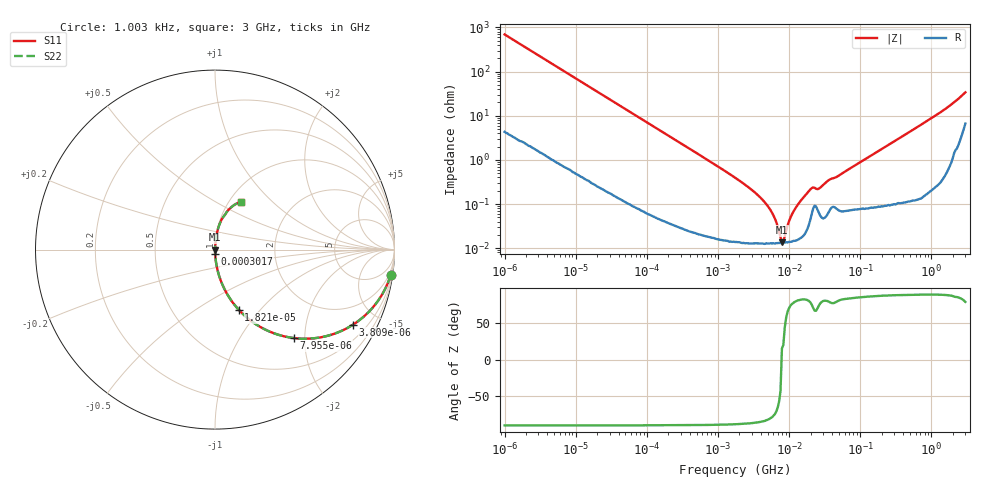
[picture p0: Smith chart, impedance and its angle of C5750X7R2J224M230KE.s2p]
! S-Parameter Data Generated by TDK Corporation
! Copyright(C) 2022 TDK Corporation.
! All Rights Reserved.
! TDK P/N: C5750X7R2J224M230KE (Multilayer Ceramic Chip Capacitor)
! Property: C=220nF
! Size(LxWxT): 5.7x5x2.3mm
! Model Type: s2p (Touchstone File Format Version 1.0)
! Frequency: DC=Yes Start=0.00100272998679MHz Stop=3000MHz 326points Log-sweep
! Model Generated on Apr. 15, 2022
! Port Assignments:
!  1 ---| |--- 2
! Applicable Conditions:
!  Temperature = 25 degC
!  DC Bias Voltage = 0 V
!  Small Signal Operation
! Terms and conditions regarding TDK Simulation Models
! (1)This simulation model is being provided solely for informational purposes. Please refer to the specifications of the products in terms of detailed characteristics of such products.
! (2)In no event shall TDK Corporation of any of its subsidiaries be liable for any loss or damage arising, directly or indirectly,
!  From any information contained in this simulation model, including, but not limited to loss or damages arising from any inaccuracies, omissions or errors in connection with such information.
! (3)Any and all copyrights on this simulation model are owned by TDK Corporation.
!  Duplication or redistribution of this simulation model without prior written permission from TDK Corporation is prohibited.
! (4)This simulation model is subject to any modification or change without any prior notice.
! (5)Neither TDK Corporation nor any of its subsidiaries shall make any warranty, express or implied,
!  Including but not limited to the correctness, implied warranties of merchantability and fitness for a particular purpose with respect to this simulation models.
! (6)The use of this simulation model shall be deemed to have consented to the terms and conditions hereof.
# Hz S MA R 50
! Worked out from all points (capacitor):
!   325 points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, 1.003 kHz to 3 GHz, reference 50 ohm
!   read as one part in series: C = 228 nF near 1.05 kHz
!   lowest |Z| = 13.5 mohm at 7.92 MHz (marker M1)
!   series resonance near 7.839 MHz, so ESL is about 1.8 nH
!   S11 on the Smith chart (normalised r, x): 1.003 kHz: 1, -14; 3.809 kHz: 1.02, -3.67; 7.955 kHz: 1.01, -1.77; 18.21 kHz: 1.01, -0.77; 301.7 kHz: 1.00, -0.05; 3 GHz: 1.13, +0.67
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1002.73  0.9889 -8.2  0.1425 81.4  0.1425 81.4  0.9889 -8.2
2094.03  0.9561 -16.7  0.2868 73.0  0.2868 73.0  0.9561 -16.7
3809.07  0.8758 -28.5  0.4767 61.1  0.4767 61.1  0.8758 -28.5
7954.6  0.6595 -48.3  0.7471 41.3  0.7471 41.3  0.6595 -48.3
12036.7  0.503 -59.4  0.8607 30.2  0.8607 30.2  0.503 -59.4
18213.5  0.36 -68.5  0.9304 21.1  0.9304 21.1  0.36 -68.5
47877.3  0.1461 -81.2  0.9881 8.4  0.9881 8.4  0.1461 -81.2
151292  0.04698 -86.8  0.9984 2.7  0.9984 2.7  0.04698 -86.8
301737  0.02364 -88.0  0.9994 1.4  0.9994 1.4  0.02364 -88.0
1816100  0.00377 -87.7  0.9999 0.2  0.9999 0.2  0.00377 -87.7
4998780  0.0009022 -81.8  0.9999 0.1  0.9999 0.1  0.0009022 -81.8
6588530  0.0003926 -70.7  0.9999 0.0  0.9999 0.0  0.0003926 -70.7
7920240  0.0001352 15.3  0.9999 -0.0  0.9999 -0.0  0.0001352 15.3
8293270  0.0001409 20.1  0.9999 -0.0  0.9999 -0.0  0.0001409 20.1
9521120  0.0003281 65.6  0.9999 -0.0  0.9999 -0.0  0.0003281 65.6
1.14456e7  0.0006679 77.3  0.9999 -0.0  0.9999 -0.0  0.0006679 77.3
2.18003e7  0.002379 70.3  0.9992 -0.1  0.9992 -0.1  0.002379 70.3
2.62067e7  0.002231 73.7  0.9994 -0.1  0.9994 -0.1  0.002231 73.7
3.6168e7  0.003493 78.8  0.9993 -0.2  0.9993 -0.2  0.003493 78.8
2.61689e8  0.02297 86.4  0.9988 -1.3  0.9988 -1.3  0.02297 86.4
1.57506e9  0.1415 80.0  0.9855 -8.1  0.9855 -8.1  0.1415 80.0
3e9  0.3039 61.4  0.8952 -17.3  0.8952 -17.3  0.3039 61.4
